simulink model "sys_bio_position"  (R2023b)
settings: Solver=FixedStepAuto  StartTime=0.0  StopTime=30  FixedStep=0.001  RelTol=1e-3
libraries: fl_lib x6, nesl_utility x2, ee_lib x1, sdl_lib x1

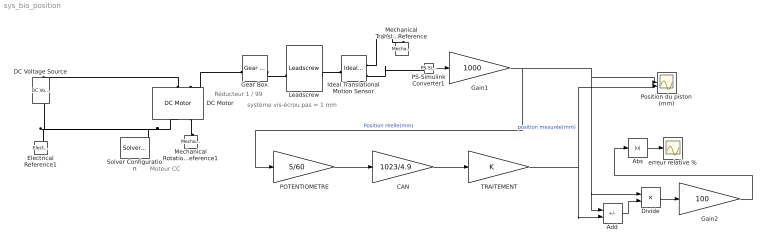
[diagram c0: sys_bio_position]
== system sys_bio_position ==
  note: système vis-écrou pas = 1 mm
  note: Moteur CC
  note: Réducteur 1 / 99
  Abs : Abs
  Add : Sum  Inputs=+-
  CAN : Gain  Gain=1023/4.9
  DC Motor : ee_lib/Electromechanical/Brushed Motors/DC Motor  field_option=ee.enum.field_option.pm  Rf=100 Ohm  Lf=1 H  Laf=0.15 H  If0=0 A  parameterization=ee.enum.dcparam_option.circuit_param  Ra=2.22 Ohm  La=0.1e-3 H  emf_or_torque=ee.enum.emf_or_torque.kv  Kv=0.0113 V/(rad/s)  Ki=0.01 N*m/A  T_stall=0.24e-3 N*m  w_max=19100 rpm  w_rated=15000 rpm  P_rated=0.08 W  V_rated=1.5 V  lam_param=ee.enum.lam_param.damping  i_noload=0 A  V_i_noload=1.5 V  J=50 g*cm^2  lam=0.0000015 N*m/(rad/s)  speed0=0 rpm  enable_fault_armature=simscape.enum.onoff.off  rev_faulted=1 / 3  G_faulted_armature=1e-5 S  fault_trigger_armature=ee.enum.faults.faultTrigger.temporal  t_fault_armature=1 s  max_permissible_current_armature=inf A  t_fail_on_current_armature=1 s  enable_fault_field=simscape.enum.onoff.off  G_faulted_field=1e-5 S  fault_trigger_field=ee.enum.faults.faultTrigger.temporal  t_fault_field=1 s  max_permissible_current_field=inf A  t_fail_on_current_field=1 s  fault_action=simscape.enum.assert.action.none  alpha=3.93e-3 1/K  Tmeas=25 degC  thermal_mass=100 J/K  initial_temperature=25 degC
  DC Voltage Source : fl_lib/Electrical/Electrical Sources/DC Voltage Source  v0=12 V
  Divide : Product  Inputs=/*
  Electrical Reference1 : fl_lib/Electrical/Electrical Elements/Electrical Reference
  Gain1 : Gain  Gain=1000
  Gain2 : Gain  Gain=100
  Gear Box : fl_lib/Mechanical/Mechanisms/Gear Box  ratio=99  t_in_specify=off  t_in_priority=None  t_in=0 N*m  t_in_nominal_specify=off  t_in_nominal_unit=N*m  t_in_nominal_value=1  t_out_specify=off  t_out_priority=None  t_out=0 N*m  t_out_nominal_specify=off  t_out_nominal_unit=N*m  t_out_nominal_value=1
  Ideal Translational Motion Sensor : fl_lib/Mechanical/Mechanical Sensors/Ideal Translational Motion Sensor  reference=foundation.enum.MeasurementReference.difference  acceleration_port=false  velocity_port=true  position_port=true  offset=0 m
  Leadscrew : sdl_lib/Gears/Rotational- Translational/Leadscrew  Lead=1 mm  helix_type=sdl.enum.handedness.right  friction_model=sdl.enum.gear_friction.constant  friction_parameterization=sdl.enum.frictionParameterization.geometry  lambda=15 deg  alpha=14.5 deg  fr_coeff=0.08  eff_sn=0.75  eff_ns=0.45  temperature_TLU=[280, 300, 320] K  efficiency_sn_TLU=[.75, .65, .6]  efficiency_ns_TLU=[.5, .45, .4]  pwr_thr=0.001 W  mu_visc=0 N*m/(rad/s)  thermal_mass=50 J/K  temperature_specify=off  temperature_priority=High  temperature=300 K  temperature_nominal_specify=off  temperature_nominal_unit=K  temperature_nominal_value=1
  Mechanical Rotational Reference1 : fl_lib/Mechanical/Rotational Elements/Mechanical Rotational Reference
  Mechanical Translational Reference : fl_lib/Mechanical/Translational Elements/Mechanical Translational Reference
  POTENTIOMETRE : Gain  Gain=5/60
  PS-Simulink Converter1 : nesl_utility/PS-Simulink Converter  PhysicalDomain=network_engine_domain  SubClassName=ps_output  LeftPortType=input  RightPortType=output  PseudoPeriodic=off  Frequencies=[]  VectorFormat=1-D array  Unit=inherit  AffineConversion=off
  Position du piston (mm) : Scope  NumInputPorts=2
  Solver Configuration : nesl_utility/Solver Configuration  PhysicalDomain=network_engine_domain  SubClassName=solver  LeftPortType=input  RightPortType=generic  Tones=[]  Harmonics=[]  SimulateNoise=off  Profile=off  UseLocalSampling=off  EnableSwitchedLinearOptims=on  FrequencyDomain=off  UseCCode=off  RelTol=0.001  AbsTol=1e-06  MinStep=1e-09  ToWorkspace=off  RevertToSquareIcSolve=off  NumHomotopyIterations=100  PhasorMode=off  PhasorModeNumHarmonics=1  ConsistencySolver=NEWTON_FTOL  IndexReductionMethod=DerivativeReplacement  DoDC=off  ResidualTolerance=1e-09  ConsistencyTolSource=GLOBAL  ConsistencyAbsTol=0.001  ConsistencyRelTol=0.001  ConsistencyTolFactor=0.001  UseLocalSolver=off  LocalSolverChoice=NE_BACKWARD_EULER_ADVANCER  ResolveIndetEquations=on  FunctionEvalNumThread=1  LocalSolverSampleTime=0.001  DoFixedCost=off  MaxNonlinIter=3  MaxModeIter=2  ComputeImpulses=off  ImpulseIterations=2  LinearAlgebra=Full  LinearAlgebraNumThread=0  EquationFormulation=NE_TIME_EF  DelaysMemoryBudget=1024  AutomaticFiltering=on  FilteringTimeConstant=0.001  PartitionStorageMethod=AS_NEEDED  PartitionMemoryBudget=1024  PartitionMethod=FAST  MultibodyUseLocalSolver=off  MultibodyLocalSolverChoice=ODE1  MultibodyLocalSolverSampleTime=0.001
  TRAITEMENT : Gain
  erreur relative % : Scope
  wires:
  PS-Simulink Converter1/1 -> Gain1/1
  Gain1/1 -> POTENTIOMETRE/1, Divide/1, Add/1, Position du piston (mm)/1  "Position réelle(mm)"
  POTENTIOMETRE/1 -> CAN/1
  CAN/1 -> TRAITEMENT/1
  TRAITEMENT/1 -> Position du piston (mm)/2, Add/2  "position mesurée(mm)"
  Add/1 -> Divide/2
  Divide/1 -> Gain2/1
  Gain2/1 -> Abs/1
  Abs/1 -> erreur relative %/1
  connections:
  Electrical Reference1/LConn1 -- DC Voltage Source/RConn1 -- DC Motor/RConn1 -- Solver Configuration/RConn1
  DC Motor/RConn2 -- Mechanical Rotational Reference1/LConn1
  Ideal Translational Motion Sensor/RConn1 -- Mechanical Translational Reference/LConn1
  Gear Box/LConn1 -- DC Motor/LConn2
  Gear Box/RConn1 -- Leadscrew/LConn1
  Leadscrew/RConn1 -- Ideal Translational Motion Sensor/LConn1
  DC Motor/LConn1 -- DC Voltage Source/LConn1
  Ideal Translational Motion Sensor/RConn3 -- PS-Simulink Converter1/LConn1
